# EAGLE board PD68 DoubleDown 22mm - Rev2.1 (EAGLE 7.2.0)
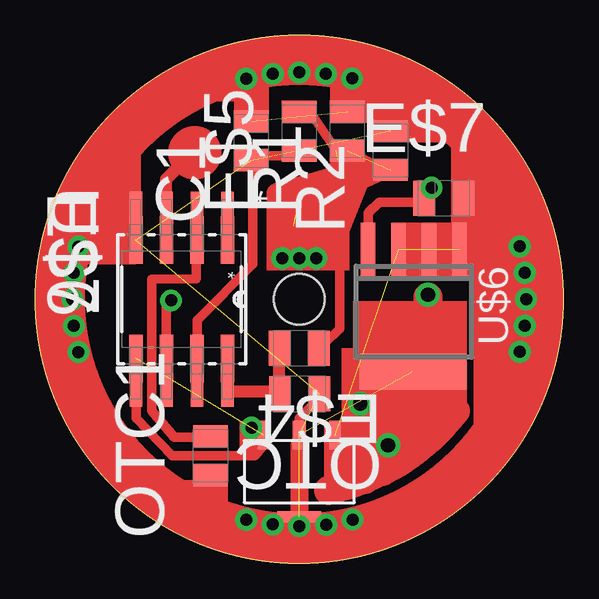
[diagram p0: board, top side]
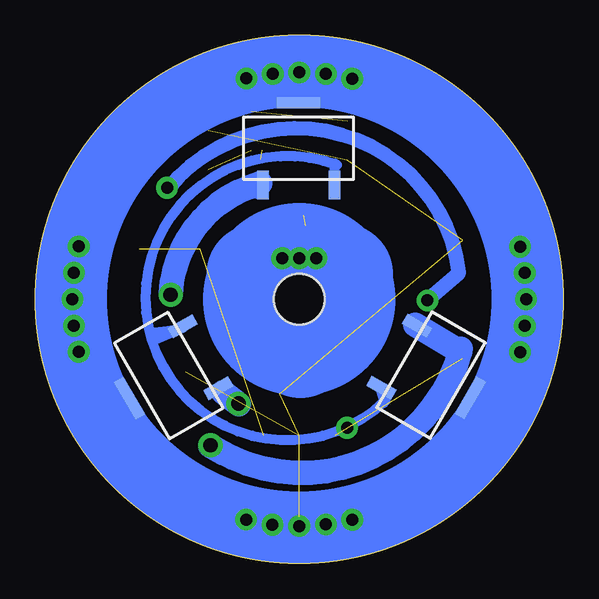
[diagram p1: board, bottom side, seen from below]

No outline drawn. Coordinates in mm, seen from the top.
Copper layers (1*16): Top 0.035mm / dielectric 1.5mm / Bottom 0.035mm
Design rules "default *": minimum track width 10mil, minimum drill 24mil, track to track 8mil, track to pad 8mil, pad to pad 8mil, via to via 8mil, smd to smd 8mil, copper to edge 40mil, drill to drill 8mil, minimum pad ring 10mil, minimum via ring 8mil, stop-mask expansion 4mil, vias tented up to drill 2500mil, thermal gap 10mil
Net classes: 0 default: clearance 0.205 mm
Holes 2.1 mm at 20,20
Milling: area 9,9 to 31,31

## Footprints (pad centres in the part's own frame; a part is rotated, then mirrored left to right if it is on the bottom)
CAPC2013X94N = smd 0.914 x 1.448: 1 -0.813,0; 2 0.813,0
AMC7135_CC_REGULATOR = smd 1.82 x 0.46: GND2 0,1.89 | smd 0.48 x 1.19: OUT -1.49,-1.525; VDD 1.49,-1.525
SOIC127P798X216-8N = smd 1.549 x 0.533: 1 -3.708,1.905; 2 -3.708,0.635; 3 -3.708,-0.635; 4 -3.708,-1.905; 5 3.708,-1.905; 6 3.708,-0.635; 7 3.708,0.635; 8 3.708,1.905
AMC7135_CC_REGULATOR' = smd 1.82 x 0.46: GND2 0,1.89 | smd 0.55 x 1.19: GND3 0,-1.525 | smd 0.48 x 1.19: OUT -1.49,-1.525; VDD 1.49,-1.525
SO8 = smd 0.6 x 2.2: 1 -1.905,-2.6; 2 -0.635,-2.6; 3 0.635,-2.6; 4 1.905,-2.6 | smd 4.425 x 1.5: 5 0.035,2.5
SOIC-8 = smd 1.981 x 0.559: 1 -2.464,1.905; 2 -2.464,0.635; 3 -2.464,-0.635; 4 -2.464,-1.905; 5 2.464,-1.905; 6 2.464,-0.635; 7 2.464,0.635; 8 2.464,1.905

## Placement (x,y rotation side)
C1  10pF  [CAPC2013X94N]  18,26.6 90 top
E$1  [AMC7135_CC_REGULATOR]  25.44,16.82 120 bottom
E$2  [AMC7135_CC_REGULATOR]  14.51,16.84 240 bottom
E$3  [AMC7135_CC_REGULATOR]  20.03,26.29 0 bottom
E$4  [CAPC2013X94N]  20,17.96 180 top
E$5  [CAPC2013X94N]  20,27 90 top
E$6  [SOIC127P798X216-8N]  15.1,20 270 top
E$7  [CAPC2013X94N]  26.02,24.21 0 top
OTC  10pF  [CAPC2013X94N]  20.01,16.06 180 top
OTC1  10pF  [CAPC2013X94N]  16.3,13.48 90 top
R1  10pF  [CAPC2013X94N]  22,27 90 top
R2  10pF  [CAPC2013X94N]  23.8,26.2 90 top
U$5  AMC7135_CC_REGULATOR  [AMC7135_CC_REGULATOR']  20,12.82 180 top
U$6  LFPAK56/SO8_FET  [SO8]  24.77,19.48 180 top
U$7  ATTINY13A-SSU  [SOIC-8]  15.1,20 270 top

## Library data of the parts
C1 OTC OTC1 R1 R2 = C_0805; MPN: 08051A100JAT2A; OC_FARNELL: 499158; OC_NEWARK: 96K4767; SUPPLIER: AVX; TOLERANCE: ±5%; VOLTAGERATING: 100V
E$1-E$3 = AMC7135_2pin
E$4 E$5 E$7 = C_0805
E$6 = Attiny85v 10SU
U$5 = AMC7135_CC_Regulator
U$6 U$7 = dan

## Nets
GROUND: C1.1 OTC.1 R2.2 U$5.GND2 U$5.GND3 U$6.5 U$7.4
LED+: C1.2 R1.2
LED-: U$5.OUT U$6.1 U$6.2 U$6.3
N$4: R1.1 R2.1
N$5: U$7.2
PWM1: U$7.6
PWM2: U$5.VDD U$7.5
VCC: U$7.8

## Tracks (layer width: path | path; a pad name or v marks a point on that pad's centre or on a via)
BATT+  (2 unrouted)
  Top 0.4: 23.49,25.16 19.84,23.5 | 21.61,25.84 19.75,23.06 | 21.54,26.21 20.45,27.8
GROUND  (6 unrouted)
LED+  (1 unrouted)
LED-  (3 unrouted)
N$4  (1 unrouted)
N$35
  Bottom 1.016: 21.63,24.83 arc-71 25.36,20.23
PWM2  (1 unrouted)
S$1
  Top 0.5: 19.15,17.8 19.15,16.15 17.05,16.15
S$2
  Bottom 0.406: 18.42,25.59 arc-244 16.41,15.77
S$3
  Bottom 1.016: 23.16,16.13 22.52,15.63
S$4
  Bottom 1.016: 13.27,17.93 arc106 23.37,13.7
S$5
  Bottom 0.4: 25.34,18.7 26.02,18.63
S$6
  Bottom 0.4: 16.48,15.67 16.25,16.08
S$7
  Top 0.4: 20.7,15.75 20,15.05 20,14.3
S$8
  Top 0.5: 14.45,24.15 14.45,25 15.4,25.95
S$9
  Bottom 1.016: 15.16,18.94 13.3,17.82
S$10
  Top 0.4: 15.7,21.75 15.7,20.85 13.85,20.84 13.85,15.35 14.8,14.25 16.3,14.25
S$11
  Top 0.4: 13.2,15.7 13.2,15.05 14.7,13.48 18.15,13.48 18.5,13.9
S$12
  Top 0.4: 22.8,21.57 22.81,21.37
S$13
  Top 0.4: 13.2,24.23 13.2,26.34 13.06,26.48
S$14
  Top 0.4: 21.52,14.71 21.97,14.71 23.46,16.2
S$15  (via drill 0.5)
  other vias: 14.66,19.95
S$16
  Top 0.4: 14.46,18.27 14.46,19.75 14.68,19.97
S$17
  Top 0.4: 18.1,29.01 18.12,27.33
S$18
  Top 0.4: 18.07,25.54 18.07,21.45 15.75,19.13 15.75,17.56 15.69,17.5
S$19
  Top 0.4: 19.6,25.99 18.31,25.99 17.92,25.6
S$20
  Top 0.4: 23.86,27.15 23.89,27.18 23.89,29.21
S$21
  Top 0.4: 21.92,27.95 21.9,29.23
S$22  (via drill 0.5)
  other vias: 25.51,24.65
S$23  (via drill 0.6)
  other vias: 25.36,20.19
S$24
  Top 0.4: 21.06,18.16 21.68,18.78 21.68,21.7 20.6,22.78 20.23,22.78
S$25  (via drill 0.6)
  other vias: 22.54,15.65
S$26  (via drill 0.6)
  other vias: 23.7,13.92
S$27
  Top 0.4: 22.88,22.87 22.88,23.6 23.33,24.05 24.87,24.05 25.41,24.59
S$28
  Top 0.4: 25.4,20.15 25.4,17.54 25.38,17.52 24.39,17.52 22.48,15.61
S$29
  Top 0.4: 24.55,14.4 24.55,16.87 23.89,16.46
S$30
  Top 0.4: 16.38,12.4 16.38,11.54
S$31  (via drill 0.5)
  other vias: 20,21.71
S$32  (via drill 0.5)
  other vias: 20.71,21.71
S$33  (via drill 0.5)
  other vias: 19.29,21.71
S$34  (via drill 0.5)
  other vias: 18.01,14.65
S$35
  Bottom 0.4: 16.65,16.38 16.48,15.82
S$36
  Bottom 0.6: 25.46,24.61 arc134 13.35,21.1
S$37
  Bottom 0.6: 13.37,21.07 14.68,19.93
S$38
  Bottom 0.406: 18.5,24.75 18.52,25.66
S$39
  Top 0.8: 23.57,25.45 20.89,24.28 22.09,25.96 23.18,25.33 22.23,25.36 19.03,24.43
S$40
  Bottom 1.016: 23.16,13.59 23.7,13.9
S$41
  Bottom 0.2: 22.22,24.51 21.72,24.26
S$42
  Top 0.8: 22.56,25.08 21.31,21.98
S$43
  Bottom 0.4: 24.85,18.8 26.02,18.29
S$44
  Top 0.4: 20,13.92 20,10.85
S$45
  Top 1.2: 26.5,15.34 arc-41 21.22,12.04
S$46
  Top 1.2: 25.36,20.09 25.36,16.41
S$47
  Top 0.75: 20,13.93 20,11.02
S$48  (via drill 0.5)
  other vias: 10.55,20
S$49  (via drill 0.5)
  other vias: 10.61,21.1
S$50  (via drill 0.5)
  other vias: 10.8,22.19
S$51  (via drill 0.5)
  other vias: 10.61,18.89
S$52  (via drill 0.5)
  other vias: 10.8,17.8
S$53  (via drill 0.5)
  other vias: 20,29.45
S$54  (via drill 0.5)
  other vias: 18.89,29.39
S$55  (via drill 0.5)
  other vias: 17.79,29.19
S$56  (via drill 0.5)
  other vias: 21.11,29.39
S$57  (via drill 0.5)
  other vias: 22.2,29.2
S$58  (via drill 0.5)
  other vias: 29.45,20
S$59  (via drill 0.5)
  other vias: 29.39,21.11
S$60  (via drill 0.5)
  other vias: 29.19,22.2
S$61  (via drill 0.5)
  other vias: 29.39,18.9
S$62  (via drill 0.5)
  other vias: 29.19,17.81
S$63  (via drill 0.5)
  other vias: 20,10.55
S$64  (via drill 0.5)
  other vias: 18.89,10.62
S$65  (via drill 0.5)
  other vias: 17.79,10.81
S$66  (via drill 0.5)
  other vias: 21.12,10.61
S$67  (via drill 0.5)
  other vias: 22.22,10.82
S$68
  Bottom 0.4: 23.62,16.14 23.36,15.9
(copper drawn outside any net)
  shapes: Bottom circle x5, Top area x18, Top circle x3

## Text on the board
tTest: Pin3 | R2 | R1 | BR | R-FET | LED+ | C1 | Rev2.1 | FET | D1 | ZNR | OTC | 7135 | LED-
bTest: DoubleDown | BLF | PD68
